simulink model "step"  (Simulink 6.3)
settings: Solver=ode3  StartTime=0.0  StopTime=200  MaxStep=.1  RelTol=1e-3

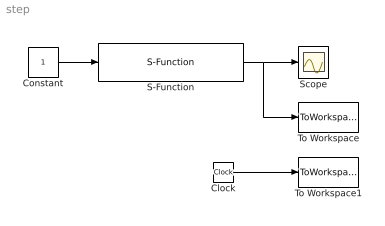
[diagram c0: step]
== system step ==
  Clock : Clock
  Constant : Constant
  S-Function : S-Function  FunctionName=sfperiodictmp  mask(prenos){b0=.120, a0=.05210, la1=0.5, la2=.4, om1=.6, om2=.1}
  Scope : Scope
  To Workspace : ToWorkspace  VariableName=simout1  SampleTime=.1  SaveFormat=Array
  To Workspace1 : ToWorkspace  VariableName=simout2  SampleTime=.1  SaveFormat=Array
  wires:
  Constant/1 -> S-Function/1
  S-Function/1 -> Scope/1, To Workspace/1
  Clock/1 -> To Workspace1/1
